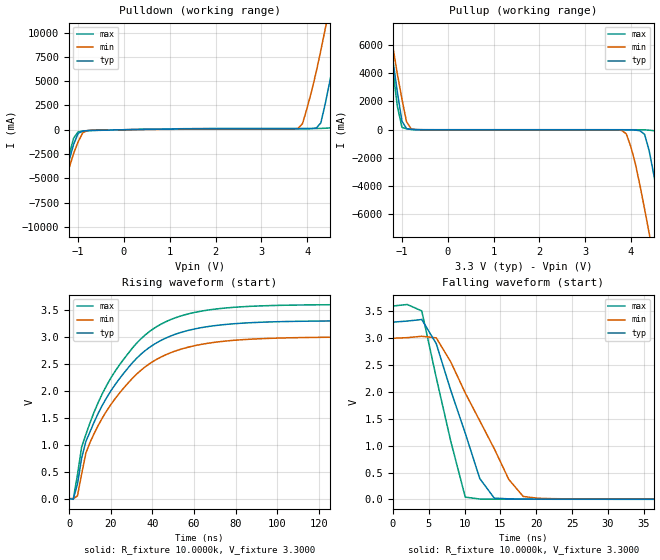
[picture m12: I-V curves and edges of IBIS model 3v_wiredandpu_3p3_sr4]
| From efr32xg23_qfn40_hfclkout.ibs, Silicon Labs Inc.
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|   Model 3v_wiredandpu_3p3_sr4
[Model]  3v_wiredandpu_3p3_sr4
Model_type Output
Polarity   Inverting
Enable   Active-Low
C_comp   1.6300pF   1.4000pF   2.7000pF
[Temperature Range]   25.0000   0.1250k   -40.0000
[Pullup Reference]   3.3000V   3.0000V   3.6000V
[Pulldown Reference]   0.0V   0.0V   0.0V
[POWER Clamp Reference]   3.3000V   3.0000V   3.6000V
[GND Clamp Reference]   0.0V   0.0V   0.0V
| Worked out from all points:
|   slope of the pulldown table from 0 to 0.495 V, typ, clamps not added: 12.7 ohm
|   slope of the pullup table from 0 to 0.495 V, typ, clamps not added: 44.2 kohm
|   rising waveform, R_fixture 10.0000k, V_fixture 3.3000: 20-80 % time 27.8ns typ, 28.3ns min, 27.3ns max; typ from 0.004 V to 3.3 V
|   falling waveform, R_fixture 10.0000k, V_fixture 3.3000: 20-80 % time 4.81ns typ, 6.71ns min, 3.72ns max; typ from 3.3 V to 0.004 V
[Pulldown]
|Voltage   I(typ)   I(min)   I(max)
-3.3V     -36.83A    -34.38A    -38.93A
-1.6V     -10.64A    -10.81A    -10.62A
-1V       -371.1mA   -1.224A    -213.8mA
-700mV    -62.65mA   -46.52mA   -78.49mA
3.8V      92.62mA    126.4mA    128.5mA
4V        98.53mA    2.235A     128.9mA
4.3V      707.5mA    8.157A     136.5mA
4.4V      2.753A     10.48A     153.5mA
4.6V      7.599A     15.23A     305.1mA
4.7V      10.27A     17.54A     1.795A
5V        18.37A     24.1A      10.26A
6.6V      55.85A     55.3A      54.07A
[Pullup]
|Voltage   I(typ)   I(min)   I(max)
-3.3V     55.71A     49.41A     61.66A
-1.3V     7.505A     8.098A     7.139A
-1.1V     2.66A      3.943A     1.662A
-900mV    80.58mA    570.7mA    64.28mA
3.8V      -800.8uA   -47.13mA   -99.31uA
4V        -7.56mA    -1.209A    -145.9uA
4.3V      -326.4mA   -5.611A    -8.338mA
4.4V      -1.482A    -7.33A     -28.81mA
4.6V      -4.973A    -10.8A     -136.7mA
4.7V      -6.847A    -12.49A    -837.2mA
5.1V      -14.25A    -18.59A    -8.585A
6.6V      -36.82A    -38.16A    -34.3A
[Ramp]
| variable   typ   min   max
dV/dt_r  0.3648/16.2447n   0.2963/17.0953n   0.4475/15.4772n
dV/dt_f  1.9778/4.8083n   1.7970/6.7107n   2.1582/3.7210n
R_load = 10.0000k
[Rising Waveform]
R_fixture= 10.0000k
V_fixture= 3.3000
V_fixture_min= 3.0000
V_fixture_max= 3.6000
|time   V(typ)   V(min)   V(max)
0s        3.603mV    4.877mV    2.979mV
2.02ns    -9.73mV    919.3uV    -10.88mV
4.04ns    270.8mV    52.21mV    441.7mV
6.061ns   752.7mV    460.2mV    961.1mV
8.081ns   1.061V     846.9mV    1.189V
18.18ns   1.881V     1.637V     2.11V
32.32ns   2.598V     2.305V     2.877V
46.46ns   2.978V     2.669V     3.28V
84.85ns   3.258V     2.952V     3.562V
200ns     3.3V       2.999V     3.6V
[Falling Waveform]
R_fixture= 10.0000k
V_fixture= 3.3000
V_fixture_min= 3.0000
V_fixture_max= 3.6000
|time   V(typ)   V(min)   V(max)
0s        3.3V       3V         3.6V
4.04ns    3.349V     3.037V     3.509V
6.061ns   2.898V     3.007V     2.266V
10.1ns    1.233V     1.981V     43.96mV
12.12ns   390mV      1.464V     8.849mV
14.14ns   25.54mV    944.4mV    6.21mV
16.16ns   11.63mV    373.7mV    5.273mV
18.18ns   8.472mV    56mV       4.802mV
20.2ns    7.124mV    23.1mV     4.522mV
200ns     3.604mV    4.88mV     2.98mV
